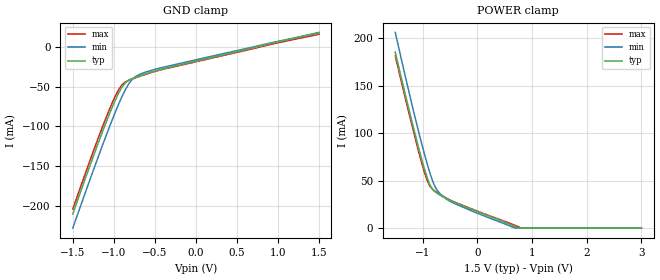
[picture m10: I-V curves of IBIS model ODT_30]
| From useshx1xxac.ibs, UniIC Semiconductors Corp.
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|   Model ODT_30
[Model]  ODT_30
Model_type   Input
Polarity   Non-Inverting
Vinl =   0.600000V
Vinh =   0.900000V
C_comp   1.3900pF   1.3640pF   1.5600pF
[Temperature Range]   25.0000   95.0000   0.0
[Voltage Range]   1.5000V   1.4000V   1.6000V
[GND_clamp]
|Voltage   I(typ)   I(min)   I(max)
-1.5V     -210.1mA   -227.8mA   -203.8mA
-1.18V    -118.2mA   -135.6mA   -112mA
-1.06V    -86.15mA   -102.6mA   -80.34mA
-980mV    -66.61mA   -81.68mA   -61.53mA
-940mV    -57.98mA   -71.8mA    -53.69mA
-900mV    -50.72mA   -62.52mA   -47.79mA
-860mV    -45.45mA   -54.11mA   -44.2mA
-780mV    -40.22mA   -41.5mA    -40.53mA
-740mV    -38.61mA   -37.82mA   -39.08mA
-620mV    -34.31mA   -32.13mA   -34.93mA
-420mV    -28.12mA   -26.33mA   -28.86mA
1.5V      17.42mA    18.09mA    15.7mA
[POWER_clamp]
|Voltage   I(typ)   I(min)   I(max)
-1.5V     185.5mA    206.3mA    181.7mA
-1.16V    104.2mA    121.9mA    100.4mA
-1.02V    73.22mA    89.76mA    69.51mA
-940mV    57.31mA    72.56mA    54.11mA
-860mV    45mA       56.97mA    43.67mA
-780mV    38.83mA    44.7mA     39.17mA
-700mV    35.46mA    37.49mA    36.14mA
-600mV    32.08mA    32.13mA    32.76mA
-460mV    28.29mA    27.13mA    28.61mA
-20mV     17.88mA    16.17mA    18.37mA
752.7mV   0A         NA         NA
3V        0A         0A         0A
